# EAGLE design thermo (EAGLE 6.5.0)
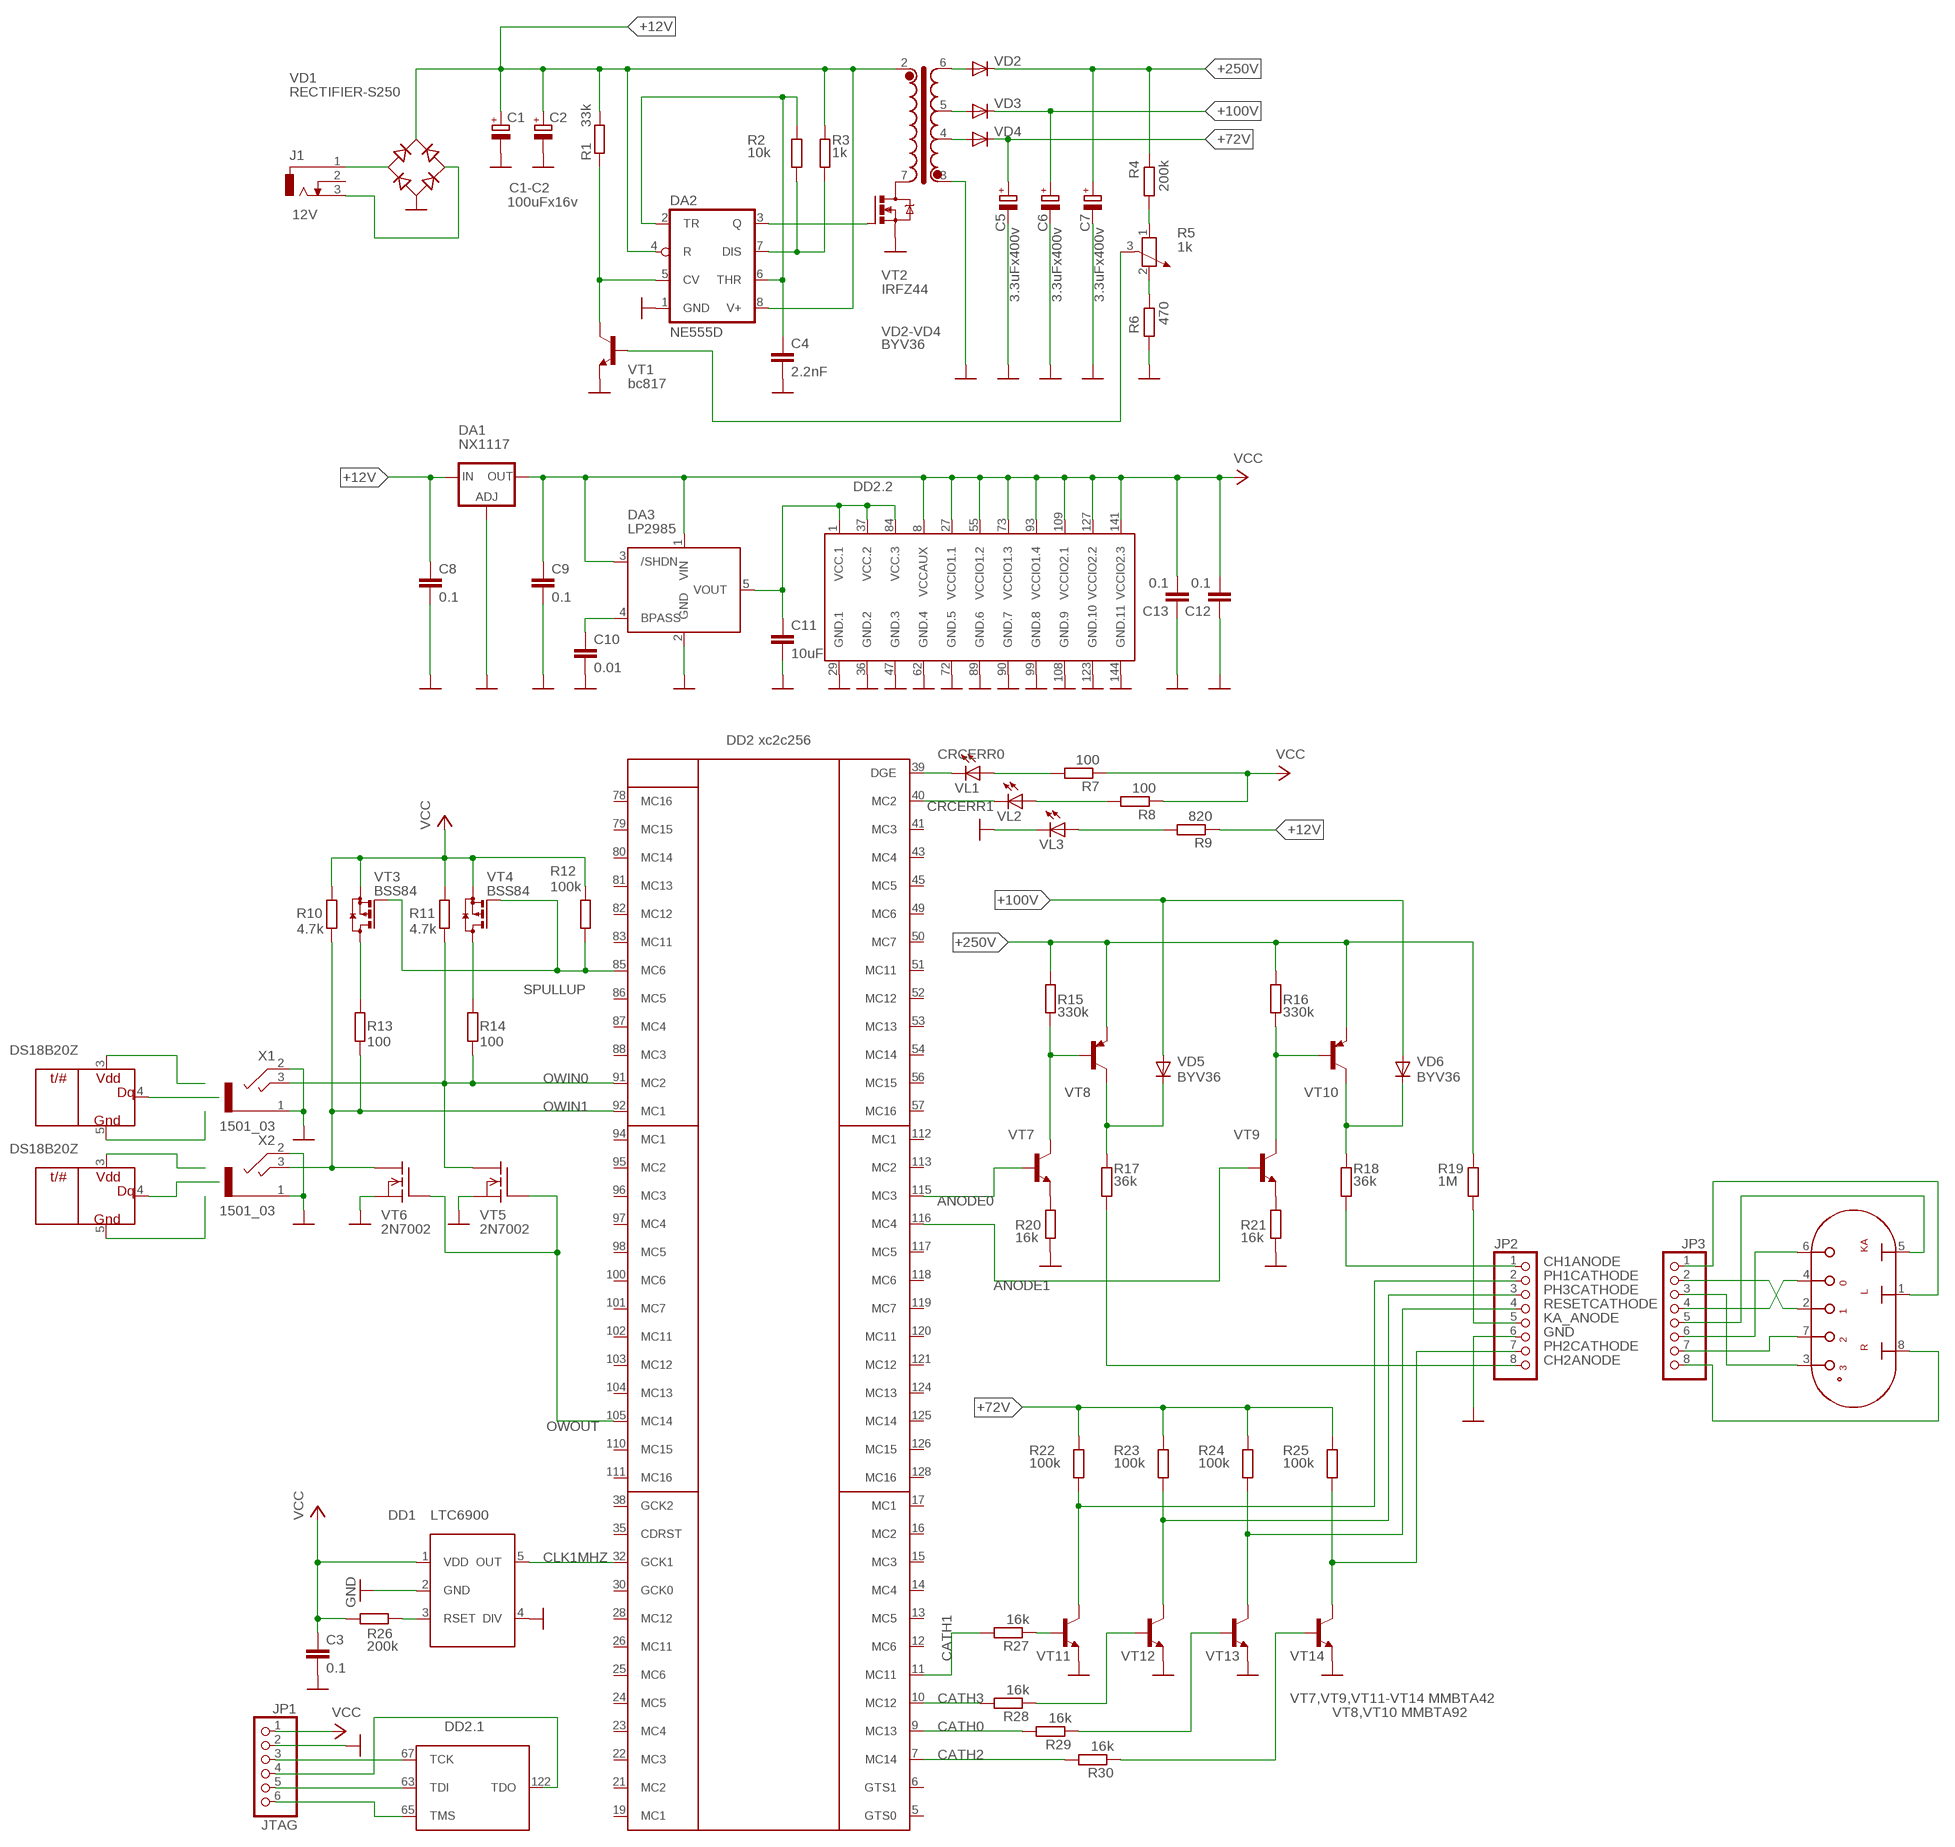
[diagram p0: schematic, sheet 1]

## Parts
C1  100uFx16v  CPOL-EUD  [PANASONIC_D]
C2  100uFx16v  CPOL-EUD  [PANASONIC_D]
C3  0.1  C-EUC1206  [C1206]
C4  2.2nF  C-EUC1206  [C1206]
C5  3.3uFx400v  CPOL-EUE5-10.5  [E5-10,5]
C6  3.3uFx400v  CPOL-EUE5-10.5  [E5-10,5]
C7  3.3uFx400v  CPOL-EUE5-10.5  [E5-10,5]
C8  0.1  C-EUC1206  [C1206]
C9  0.1  C-EUC1206  [C1206]
C10  0.01  C-EUC1206  [C1206]
C11  10uF  C-EUC1206  [C1206]
C12  0.1  C-EUC1206  [C1206]
C13  0.1  C-EUC1206  [C1206]
DA1  NX1117  LD117AS33TR  [SOT223]
DA2  NE555D  [SO08]
DA3  LP2985  [SOT23-5]
DD1  LTC6900  [SOT23-5]
DD2  XC2C128  [TQ144]
J1  DCJ0303  [DCJ0303]
JP1  PINHD-1X6  [1X06]
JP2  PINHD-1X8  [1X08]
JP3  PINHD-1X8  [1X08]
R1  33k  R-EU_R1206  [R1206]
R2  10k  R-EU_R1206  [R1206]
R3  1k  R-EU_R1206  [R1206]
R4  200k  R-EU_R1206  [R1206]
R5  1k  POTENTIOMETER_PT-10  [PT-10]
R6  470  R-EU_R1206  [R1206]
R7  100  R-EU_R1206  [R1206]
R8  100  R-EU_R1206  [R1206]
R9  820  R-EU_R1206  [R1206]
R10  4.7k  R-EU_R1206  [R1206]
R11  4.7k  R-EU_R1206  [R1206]
R12  100k  R-EU_R1206  [R1206]
R13  100  R-EU_R1206  [R1206]
R14  100  R-EU_R1206  [R1206]
R15  330k  R-EU_R1206  [R1206]
R16  330k  R-EU_R1206  [R1206]
R17  36k  R-EU_R1206  [R1206]
R18  36k  R-EU_R1206  [R1206]
R19  1M  R-EU_R1206  [R1206]
R20  16k  R-EU_R1206  [R1206]
R21  16k  R-EU_R1206  [R1206]
R22  100k  R-EU_R1206  [R1206]
R23  100k  R-EU_R1206  [R1206]
R24  100k  R-EU_R1206  [R1206]
R25  100k  R-EU_R1206  [R1206]
R26  200k  R-EU_R1206  [R1206]
R27  16k  R-EU_R1206  [R1206]
R28  16k  R-EU_R1206  [R1206]
R29  16k  R-EU_R1206  [R1206]
R30  16k  R-EU_R1206  [R1206]
T1  TRANSFORM-1  [EFD20-8]
U$2  BG12201  [BG12201]
U$3  DS18B20Z  [SO08]
U$4  DS18B20Z  [SO08]
VD1  RECTIFIER-S250  [TO-269AA]
VD2  BYV36  [SOD57-10]
VD3  BYV36  [SOD57-10]
VD4  BYV36  [SOD57-10]
VD5  BYV36  [SOD57-10]
VD6  BYV36  [SOD57-10]
VL1  LEDCHIPLED_0805  [CHIPLED_0805]
VL2  LEDCHIPLED_0805  [CHIPLED_0805]
VL3  LEDCHIPLED_0805  [CHIPLED_0805]
VT1  bc817  MMBTA42LT1-NPN-SOT23-BEC  [SOT23-BEC]
VT2  IRFZ44  IRFZ48Z  [TO220BH]
VT3  BSS84  [SOT23]
VT4  BSS84  [SOT23]
VT5  2N7002  [SOT23]
VT6  2N7002  [SOT23]
VT7  mmbta42  MMBTA42LT1-NPN-SOT23-BEC  [SOT23-BEC]
VT8  mmbta92  MMBTA92LT1-PNP-SOT23-BEC  [SOT23-BEC]
VT9  mmbta42  MMBTA42LT1-NPN-SOT23-BEC  [SOT23-BEC]
VT10  mmbta92  MMBTA92LT1-PNP-SOT23-BEC  [SOT23-BEC]
VT11  mmbta42  MMBTA42LT1-NPN-SOT23-BEC  [SOT23-BEC]
VT12  mmbta42  MMBTA42LT1-NPN-SOT23-BEC  [SOT23-BEC]
VT13  mmbta42  MMBTA42LT1-NPN-SOT23-BEC  [SOT23-BEC]
VT14  mmbta42  MMBTA42LT1-NPN-SOT23-BEC  [SOT23-BEC]
X1  1501_03  [1501_03]
X2  1501_03  [1501_03]

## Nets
+12V: C1.+ C2.+ C8.1 DA1.3(IN) DA2.4(R) DA2.8(V+) R1.1 R3.1 R9.1 T1.2 VD1.+
+72V: C5.+ R22.2 R23.2 R24.2 R25.2 VD4.C
+100V: C6.+ VD3.C VD5.A VD6.A
+250V: C7.+ R4.1 R15.2 R16.2 R19.2 VD2.C VT8.E VT10.E
ANODE0: DD2.115(FB7:MC3) VT7.B
ANODE1: DD2.116(FB7:MC4) VT9.B
CATH0: DD2.9(FB1:MC13) R29.2
CATH1: DD2.11(FB1:MC11) R27.2
CATH2: DD2.7(FB1:MC14) R30.2
CATH3: DD2.10(FB1:MC12) R28.2
CH1ANODE: JP2.1 R18.1
CH2ANODE: JP2.8 R17.1
CLK1MHZ: DD1.5(OUT) DD2.32(FB2:GCK1)
CRCERR0: DD2.39(FB4:DGE) VL1.C
CRCERR1: DD2.40(FB4:MC2) VL2.C
GND: C1.- C2.- C3.2 C4.2 C5.- C6.- C7.- C8.2 C9.2 C10.2 C11.2 C12.1 C13.1 DA1.1(ADJ) DA2.1(GND) DA3.2(GND) DD1.2(GND) DD1.4(DIV) DD2.29(PWR:GND.1) DD2.36(PWR:GND.2) DD2.47(PWR:GND.3) DD2.62(PWR:GND.4) DD2.72(PWR:GND.5) DD2.89(PWR:GND.6) DD2.90(PWR:GND.7) DD2.99(PWR:GND.8) DD2.108(PWR:GND.9) DD2.123(PWR:GND.10) DD2.144(PWR:GND.11) JP1.2 JP2.6 R6.2 R20.1 R21.1 T1.3 VD1.- VL3.C VT1.E VT2.S VT5.2(S) VT6.2(S) VT11.E VT12.E VT13.E VT14.E X1.1 X1.2 X2.1 X2.2
KA_ANODE: JP2.5 R19.1
N$1: DD1.3(RSET) R26.1
N$2: JP3.1 U$2.1(LA)
N$3: JP3.2 U$2.2(C1)
N$4: C11.1 DA3.5(VOUT) DD2.1(PWR:VCC.1) DD2.37(PWR:VCC.2) DD2.84(PWR:VCC.3)
N$5: JP3.3 U$2.3(C3)
N$6: C10.1 DA3.4(BPASS)
N$7: R20.2 VT7.E
N$8: R21.2 VT9.E
N$9: R15.1 VT7.C VT8.B
N$10: DA2.3(Q) VT2.G
N$11: R16.1 VT9.C VT10.B
N$12: JP3.4 U$2.4(CR)
N$13: JP3.5 U$2.5(KA_A)
N$14: JP3.6 U$2.6(KA_C)
N$15: JP3.7 U$2.7(C2)
N$16: T1.7 VT2.D
N$17: R27.1 VT11.B
N$18: R28.1 VT12.B
N$19: R29.1 VT13.B
N$20: R30.1 VT14.B
N$21: R17.2 VD5.C VT8.C
N$22: R18.2 VD6.C VT10.C
N$23: C4.1 DA2.2(TR) DA2.6(THR) R2.1
N$24: DA2.7(DIS) R2.2 R3.2
N$25: R14.2 VT4.3(D)
N$26: T1.6 VD2.A
N$27: DA2.5(CV) R1.2 VT1.C
N$28: R5.3 VT1.B
N$29: T1.5 VD3.A
N$30: T1.4 VD4.A
N$31: JP3.8 U$2.8(RA)
N$32: U$4.4(DQ)
N$33: U$4.3(VDD)
N$34: DD2.67(JTAG:TCK) JP1.3
N$35: DD2.122(JTAG:TDO) JP1.4
N$36: DD2.63(JTAG:TDI) JP1.5
N$37: DD2.65(JTAG:TMS) JP1.6
N$38: R5.2 R6.1
N$39: R4.2 R5.1
N$40: U$4.5(GND)
N$41: U$3.5(GND)
N$42: J1.1 VD1.AC1
N$43: J1.3 VD1.AC2
N$44: R13.2 VT3.3(D)
N$45: U$3.4(DQ)
N$46: U$3.3(VDD)
N$53: R7.2 VL1.A
N$54: R8.2 VL2.A
N$56: R9.2 VL3.A
OWIN0: DD2.91(FB6:MC2) R11.1 R14.1 VT5.3(D) X1.3
OWIN1: DD2.92(FB6:MC1) R10.1 R13.1 VT6.3(D) X2.3
OWOUT: DD2.105(FB5:MC14) VT5.1(G) VT6.1(G)
PH1CATHODE: JP2.2 R22.1 VT11.C
PH2CATHODE: JP2.7 R25.1 VT14.C
PH3CATHODE: JP2.3 R23.1 VT12.C
RESETCATHODE: JP2.4 R24.1 VT13.C
SPULLUP: DD2.85(FB6:MC6) R12.1 VT3.1(G) VT4.1(G)
VCC: C3.1 C9.1 C12.2 C13.2 DA1.4(OUT) DA3.1(VIN) DA3.3(/SHDN) DD1.1(VDD) DD2.8(PWR:VCCAUX) DD2.27(PWR:VCCIO1.1) DD2.55(PWR:VCCIO1.2) DD2.73(PWR:VCCIO1.3) DD2.93(PWR:VCCIO1.4) DD2.109(PWR:VCCIO2.1) DD2.127(PWR:VCCIO2.2) DD2.141(PWR:VCCIO2.3) JP1.1 R7.1 R8.1 R10.2 R11.2 R12.2 R26.2 VT3.2(S) VT4.2(S)
Unconnected: DD2.2(FB3:GTS2) DD2.3(FB3:GTS3) DD2.4(FB3:MC1) DD2.5(FB1:GTS0) DD2.6(FB1:GTS1) DD2.12(FB1:MC6) DD2.13(FB1:MC5) DD2.14(FB1:MC4) DD2.15(FB1:MC3) DD2.16(FB1:MC2) DD2.17(FB1:MC1) DD2.19(FB2:MC1) DD2.21(FB2:MC2) DD2.22(FB2:MC3) DD2.23(FB2:MC4) DD2.24(FB2:MC5) DD2.25(FB2:MC6) DD2.26(FB2:MC11) DD2.28(FB2:MC12) DD2.30(FB2:GCK0) DD2.35(FB2:CDRST) DD2.38(FB2:GCK2) DD2.41(FB4:MC3) DD2.43(FB4:MC4) DD2.45(FB4:MC5) DD2.49(FB4:MC6) DD2.50(FB4:MC7) DD2.51(FB4:MC11) DD2.52(FB4:MC12) DD2.53(FB4:MC13) DD2.54(FB4:MC14) DD2.56(FB4:MC15) DD2.57(FB4:MC16) DD2.58(FB8:MC16) DD2.59(FB8:MC15) DD2.60(FB8:MC14) DD2.61(FB8:MC13) DD2.64(FB8:MC12) DD2.68(FB8:MC11) DD2.69(FB8:MC6) DD2.70(FB8:MC5) DD2.71(FB8:MC4) DD2.74(FB8:MC3) DD2.76(FB8:MC2) DD2.77(FB8:MC1) DD2.78(FB6:MC16) DD2.79(FB6:MC15) DD2.80(FB6:MC14) DD2.81(FB6:MC13) DD2.82(FB6:MC12) DD2.83(FB6:MC11) DD2.86(FB6:MC5) DD2.87(FB6:MC4) DD2.88(FB6:MC3) DD2.94(FB5:MC1) DD2.95(FB5:MC2) DD2.96(FB5:MC3) DD2.97(FB5:MC4) DD2.98(FB5:MC5) DD2.100(FB5:MC6) DD2.101(FB5:MC7) DD2.102(FB5:MC11) DD2.103(FB5:MC12) DD2.104(FB5:MC13) DD2.110(FB5:MC15) DD2.111(FB5:MC16) DD2.112(FB7:MC1) DD2.113(FB7:MC2) DD2.117(FB7:MC5) DD2.118(FB7:MC6) DD2.119(FB7:MC7) DD2.120(FB7:MC11) DD2.121(FB7:MC12) DD2.124(FB7:MC13) DD2.125(FB7:MC14) DD2.126(FB7:MC15) DD2.128(FB7:MC16) DD2.129(FB3:MC16) DD2.130(FB3:MC15) DD2.131(FB3:MC14) DD2.132(FB3:MC13) DD2.133(FB3:MC12) DD2.134(FB3:MC11) DD2.136(FB3:MC7) DD2.138(FB3:MC6) DD2.140(FB3:MC5) DD2.143(FB3:GSR) J1.2

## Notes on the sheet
- C1-C2
- 12V
- VD2-VD4
- DD2.2
- DD2 xc2c256
- DD1 | LTC6900
- VT7,VT9,VT11-VT14 MMBTA42
- VT8,VT10 MMBTA92
- DD2.1
- JTAG

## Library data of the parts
C1 C2 C5-C7 = rcl:CPOL-EU: POLARIZED CAPACITOR, European symbol
C3 C4 C8-C10 C12 C13 = rcl:C-EU: CAPACITOR, European symbol
C11 = rcl:C-EU: CAPACITOR, European symbol; ESR: 10-20mOhm
DA1 = v-reg:LD117A?*: Low drop fixed and adjustable positive voltage regulators 1 A Source: http://www.st.com/stonline/products/literature/ds/7194/ld1117axx.pdf
DA2 = linear:*555: TIMER
DA3 = coolrunner:LP2985
DD1 = coolrunner:LTC6900
DD2 = coolrunner:XC2C128
J1 = con-jack:DCJ0303: DC POWER JACK Source: DCJ0303.pdf; OC_FARNELL: unknown; OC_NEWARK: unknown
JP1 = pinhead:PINHD-1X6: PIN HEADER
JP2 JP3 = pinhead:PINHD-1X8: PIN HEADER
R1-R4 R6-R30 = rcl:R-EU_: RESISTOR, European symbol
R5 = rcl:POTENTIOMETER_: Potentiometer
T1 = nixie_term:TRANSFORM
U$2 = nixie_term:BG12201
U$3 U$4 = nixie_term:DS18B20
VD1 = rectifier:RECTIFIER-: Rectifier
VD2-VD6 = diode:BYV36: DIODE
VL1-VL3 = led:LED: LED
VT1 VT7 VT9 VT11-VT14 = transistor-neu-to92:*-NPN-: NPN Transistror
VT2 = transistor-power:IRFZ48: N Channel HEXFET® Power MOSFET Logic Level Source: http://www.irf.com/product-info/datasheets/data/irfz48z.pdf
VT3 VT4 = transistor-small-signal:BSS84: P-CHANNEL MOS FET
VT5 VT6 = battery:2N7002
VT8 VT10 = transistor-neu-to92:*-PNP-: PNP Transistror
X1 X2 = con-lumberg:1501_03: Klinkensteckverbinder nach JISC 6560, 2,5 mm Jack connectors according to JISC 6560, 2.5 mm Source: http://www.lumberg.com/Produkte/PDFs/1501_03.pdf; OC_FARNELL: 1200127; OC_NEWARK: unknown

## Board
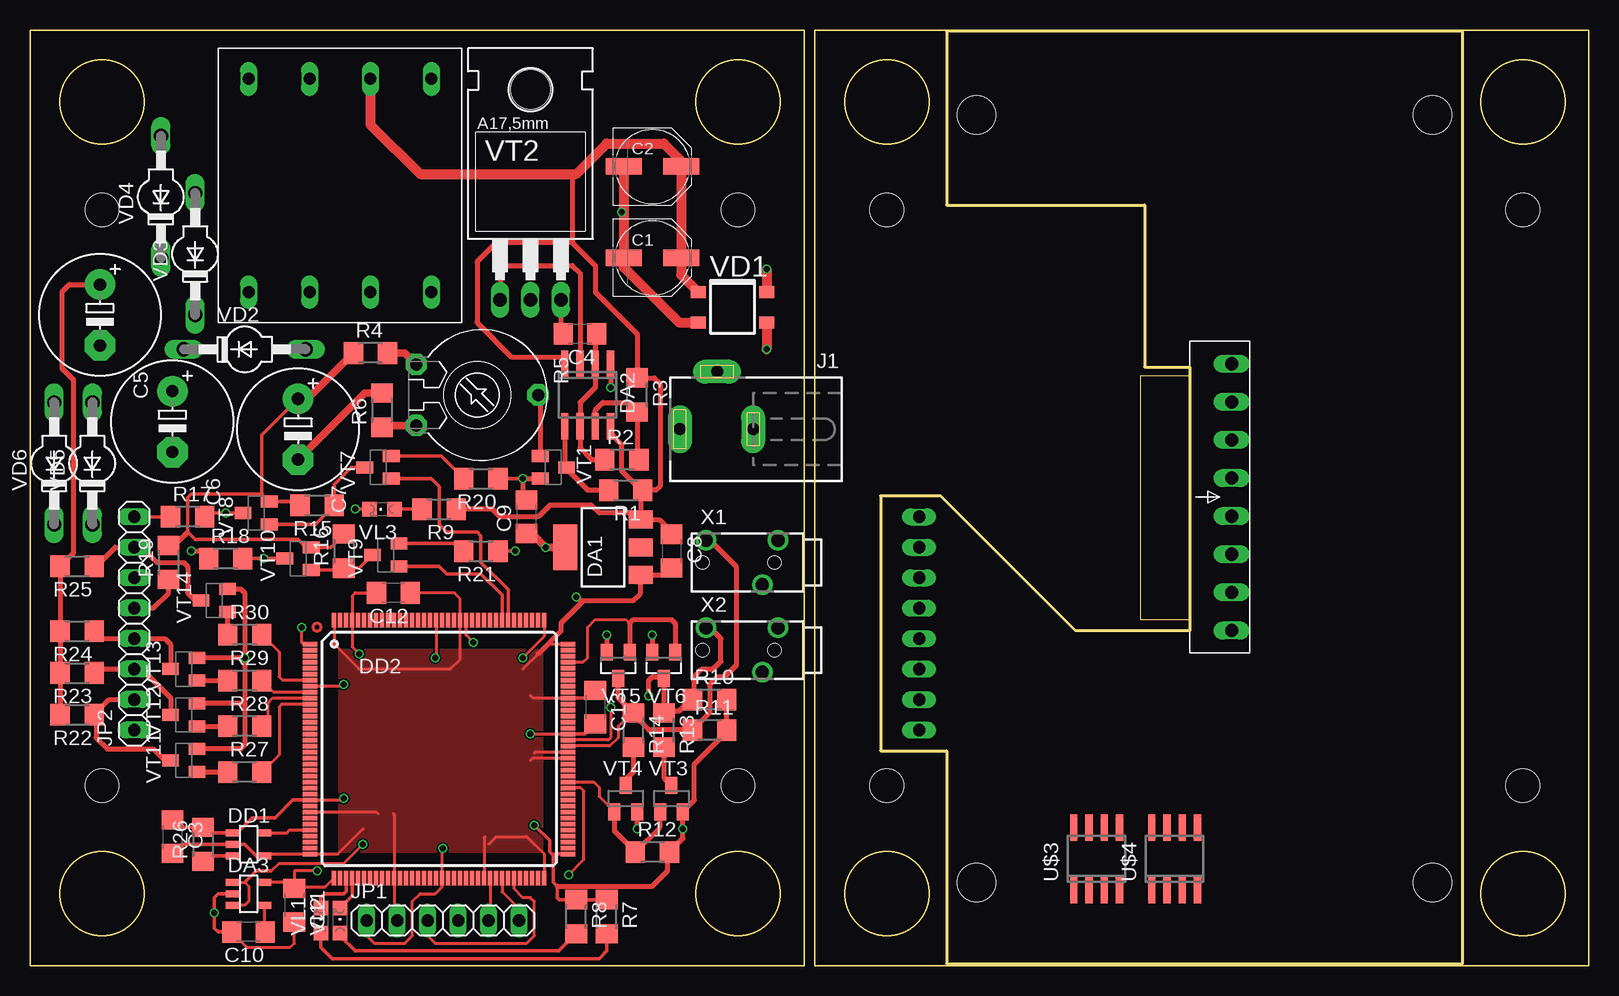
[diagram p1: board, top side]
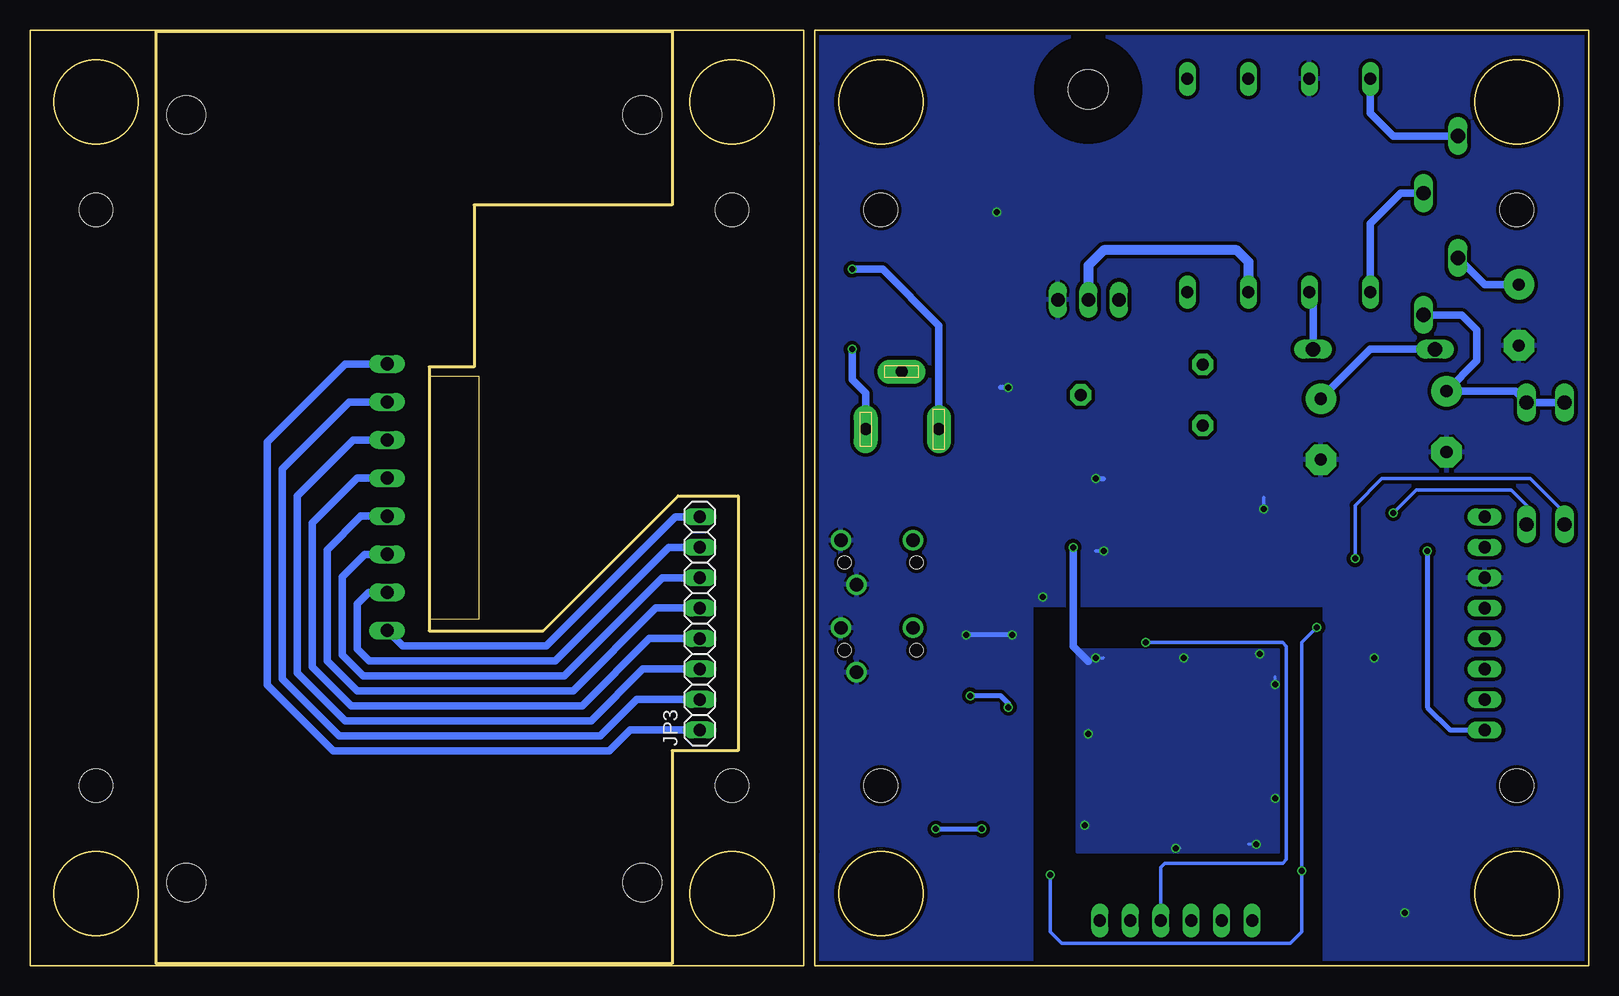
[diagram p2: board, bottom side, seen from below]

Size 129.9 x 78 mm. Coordinates in mm from the lower left corner, seen from the top.
Outline: 70.89,39.15 70.89,17.9 76.39,17.9 76.39,0.15 119.39,0.15 119.39,77.9 76.39,77.9 76.39,63.4 92.89,63.4 92.89,49.9 96.64,49.9 96.64,27.9 87.14,27.9 75.89,39.15 70.89,39.15
Copper layers (1*16): Top 0.035mm / dielectric 1.5mm / Bottom 0.035mm
Design rules "PCB-POOL HighSpec *": minimum track width 0.125mm, minimum drill 0.2mm, track to track 0.125mm, track to pad 0.125mm, pad to pad 0.125mm, via to via 0.125mm, smd to smd 0.125mm, copper to edge 0.3mm, drill to drill 0.2mm, minimum pad ring 0.2mm, minimum via ring 0.125mm, stop-mask expansion 0.075mm, vias tented up to drill 0mil, thermal gap 0.2mm
Holes 3.2 mm at 116.89,70.9 78.89,70.9 78.89,6.9 116.89,6.9

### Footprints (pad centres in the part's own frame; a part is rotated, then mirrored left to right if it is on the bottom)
PANASONIC_D = smd 3 x 1.4: + 2.4,0; - -2.4,0
C1206 = smd 1.6 x 1.8: 1 -1.4,0; 2 1.4,0
E5-10,5 = drill 1.016 pad 2.54: + -2.54,0 | drill 1.016 pad 2.54 octagon: - 2.54,0
SOT223 = smd 1.5 x 2: 1 -2.3,-3.15; 2 0,-3.15; 3 2.3,-3.15 | smd 3.8 x 2: 4 0,3.15
SO08 = smd 0.6 x 2.2: 1 -1.905,-2.6; 2 -0.635,-2.6; 3 0.635,-2.6; 4 1.905,-2.6; 5 1.905,2.6; 6 0.635,2.6; 7 -0.635,2.6; 8 -1.905,2.6
SOT23-5 = smd 0.6 x 1.2: 1 -0.95,-1.306; 2 0,-1.306; 3 0.95,-1.306; 4 0.95,1.306; 5 -0.95,1.306
TQ144 = smd 1.2 x 0.35: 1 -10.75,8.75; 2 -10.75,8.25; 3 -10.75,7.75; 4 -10.75,7.25; 5 -10.75,6.75; 6 -10.75,6.25; 7 -10.75,5.75; 8 -10.75,5.25; 9 -10.75,4.75; 10 -10.75,4.25; 11 -10.75,3.75; 12 -10.75,3.25; 13 -10.75,2.75; 14 -10.75,2.25; 15 -10.75,1.75; 16 -10.75,1.25; 17 -10.75,0.75; 18 -10.75,0.25; 19 -10.75,-0.25; 20 -10.75,-0.75; 21 -10.75,-1.25; 22 -10.75,-1.75; 23 -10.75,-2.25; 24 -10.75,-2.75; 25 -10.75,-3.25; 26 -10.75,-3.75; 27 -10.75,-4.25; 28 -10.75,-4.75; 29 -10.75,-5.25; 30 -10.75,-5.75; 31 -10.75,-6.25; 32 -10.75,-6.75; 33 -10.75,-7.25; 34 -10.75,-7.75; 35 -10.75,-8.25; 36 -10.75,-8.75; 73 10.75,-8.75; 74 10.75,-8.25; 75 10.75,-7.75; 76 10.75,-7.25; 77 10.75,-6.75; 78 10.75,-6.25; 79 10.75,-5.75; 80 10.75,-5.25; 81 10.75,-4.75; 82 10.75,-4.25; 83 10.75,-3.75; 84 10.75,-3.25; 85 10.75,-2.75; 86 10.75,-2.25; 87 10.75,-1.75; 88 10.75,-1.25; 89 10.75,-0.75; 90 10.75,-0.25; 91 10.75,0.25; 92 10.75,0.75; 93 10.75,1.25; 94 10.75,1.75; 95 10.75,2.25; 96 10.75,2.75; 97 10.75,3.25; 98 10.75,3.75; 99 10.75,4.25; 100 10.75,4.75; 101 10.75,5.25; 102 10.75,5.75; 103 10.75,6.25; 104 10.75,6.75; 105 10.75,7.25; 106 10.75,7.75; 107 10.75,8.25; 108 10.75,8.75 | smd 0.35 x 1.2: 37 -8.75,-10.75; 38 -8.25,-10.75; 39 -7.75,-10.75; 40 -7.25,-10.75; 41 -6.75,-10.75; 42 -6.25,-10.75; 43 -5.75,-10.75; 44 -5.25,-10.75; 45 -4.75,-10.75; 46 -4.25,-10.75; 47 -3.75,-10.75; 48 -3.25,-10.75; 49 -2.75,-10.75; 50 -2.25,-10.75; 51 -1.75,-10.75; 52 -1.25,-10.75; 53 -0.75,-10.75; 54 -0.25,-10.75; 55 0.25,-10.75; 56 0.75,-10.75; 57 1.25,-10.75; 58 1.75,-10.75; 59 2.25,-10.75; 60 2.75,-10.75; 61 3.25,-10.75; 62 3.75,-10.75; 63 4.25,-10.75; 64 4.75,-10.75; 65 5.25,-10.75; 66 5.75,-10.75; 67 6.25,-10.75; 68 6.75,-10.75; 69 7.25,-10.75; 70 7.75,-10.75; 71 8.25,-10.75; 72 8.75,-10.75; 109 8.75,10.75; 110 8.25,10.75; 111 7.75,10.75; 112 7.25,10.75; 113 6.75,10.75; 114 6.25,10.75; 115 5.75,10.75; 116 5.25,10.75; 117 4.75,10.75; 118 4.25,10.75; 119 3.75,10.75; 120 3.25,10.75; 121 2.75,10.75; 122 2.25,10.75; 123 1.75,10.75; 124 1.25,10.75; 125 0.75,10.75; 126 0.25,10.75; 127 -0.25,10.75; 128 -0.75,10.75; 129 -1.25,10.75; 130 -1.75,10.75; 131 -2.25,10.75; 132 -2.75,10.75; 133 -3.25,10.75; 134 -3.75,10.75; 135 -4.25,10.75; 136 -4.75,10.75; 137 -5.25,10.75; 138 -5.75,10.75; 139 -6.25,10.75; 140 -6.75,10.75; 141 -7.25,10.75; 142 -7.75,10.75; 143 -8.25,10.75; 144 -8.75,10.75
DCJ0303 = drill 1 pad 2 long: 1 0,3.1; 2 4.8,0; 3 0,-3
1X06 = drill 1.016 long: 1 -6.35,0; 2 -3.81,0; 3 -1.27,0; 4 1.27,0; 5 3.81,0; 6 6.35,0
1X08 = drill 1.016 long: 1 -8.89,0; 2 -6.35,0; 3 -3.81,0; 4 -1.27,0; 5 1.27,0; 6 3.81,0; 7 6.35,0; 8 8.89,0
R1206 = smd 1.6 x 1.803: 1 -1.422,0; 2 1.422,0
PT-10 = drill 1.016 pad 1.778 octagon: 1 -2.54,-5.08; 2 2.54,-5.08; 3 0,5.08
EFD20-8 = drill 1 long: 1 -8.89,7.62; 2 -8.89,2.54; 3 -8.89,-2.54; 4 -8.89,-7.62; 5 8.89,-7.62; 6 8.89,-2.54; 7 8.89,2.54; 8 8.89,7.62
50-200-11 = hole 2.8: -24,-26.5; 24,-26.5; 24,26.5; -24,26.5
BG12201 = drill 1.1 long: 1 11.113,0; 2 7.938,0; 3 4.763,0; 4 1.587,0; 5 -1.587,0; 6 -4.763,0; 7 -7.938,0; 8 -11.113,0
TO-269AA = smd 1 x 1.25: + -1.28,-2.855; - 1.28,-2.855; AC1 -1.28,2.855; AC2 1.28,2.855
SOD57-10 = drill 1.194 long: A 5.08,0; C -5.08,0
CHIPLED_0805 = smd 1.2 x 1.2: A 0,-1.05; C 0,1.05
SOT23-BEC = smd 1 x 1.4: B -0.95,-1.1; C 0,1.1; E 0.95,-1.1
TO220BH = drill 1.118 long: D 0,-6.35; G -2.54,-6.35; S 2.54,-6.35 | hole 3.302: 0,11.176
SOT23 = smd 1 x 1.4: 1 -0.95,-1.1; 2 0.95,-1.1; 3 0,1.1
1501_03 = drill 1.1 pad 1.7: 1 -1.85,0.3; 2 1.85,-1; 3 -1.85,-5.7 | hole 1.1: 0,0; 0,-6

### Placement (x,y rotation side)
C1  51.87,59 0 top
C2  51.87,66.62 0 top
C3  11.86,10.74 270 top
C4  45.84,52.65 180 top
C5  5.83,54.24 270 top
C6  11.86,45.35 270 top
C7  22.34,44.71 270 top
C8  53.45,34.55 270 top
C9  41.39,37.41 90 top
C10  18.21,2.8 180 top
C11  22.02,5.03 270 top
C12  30.28,31.06 180 top
C13  47.11,21.54 270 top
DA1  47.74,34.87 90 top
DA2  46.47,47.57 180 top
DA3  18.21,5.98 270 top
DD1  18.21,10.11 270 top
DD2  34.09,18.04 0 top
J1  57.27,44.71 90 top
JP1  34.41,3.76 0 top
JP2  8.69,28.52 90 top
JP3  74.09,28.52 90 bottom
R1  49.64,39.63 180 top
R2  49.33,42.17 0 top
R3  50.6,47.57 270 top
R4  28.37,51.06 0 top
R5  37.26,47.57 270 top
R6  29.33,46.3 90 top
R7  48.06,4.07 270 top
R8  45.52,4.07 270 top
R9  34.09,38.05 180 top
R10  56.63,22.17 0 top
R11  56.63,19.63 0 top
R12  51.87,9.47 0 top
R13  52.82,19.63 270 top
R14  50.28,19.63 270 top
R15  23.93,38.37 180 top
R16  26.15,34.55 90 top
R17  13.13,37.41 0 top
R18  16.31,33.92 0 top
R19  11.55,33.6 90 top
R20  37.58,40.59 180 top
R21  37.58,34.55 180 top
R22  3.93,20.9 180 top
R23  3.93,24.39 180 top
R24  3.93,27.89 180 top
R25  3.93,33.28 180 top
R26  14.4,10.11 90 top
R27  17.9,16.14 0 top
R28  17.9,19.95 0 top
R29  17.9,23.76 0 top
R30  17.9,27.57 0 top
T1  25.83,65.03 270 top
U$1  [50-200-11]  97.91,39 270 top
U$2  100.14,39.05 90 top
U$3  88.89,8.9 0 top
U$4  95.39,8.9 0 top
U$5  [50-200-11]  32.5,39 270 top
VD1  58.53,54.88 270 top
VD2  17.9,51.38 0 top
VD3  13.77,59.32 90 top
VD4  10.91,64.08 90 top
VD5  5.2,41.86 90 top
VD6  2.02,41.86 90 top
VL1  24.25,3.76 0 top
VL2  25.83,3.76 0 top
VL3  29.33,38.05 90 top
VT1  43.61,41.54 270 top
VT2  41.71,61.86 0 top
VT3  53.45,13.92 0 top
VT4  49.64,13.92 0 top
VT5  49.01,25.03 180 top
VT6  52.82,25.03 180 top
VT7  29.01,41.54 90 top
VT8  18.85,37.73 90 top
VT9  29.64,34.24 90 top
VT10  22.34,33.92 90 top
VT11  12.82,17.09 90 top
VT12  12.82,20.9 90 top
VT13  12.82,24.71 90 top
VT14  15.36,30.43 90 top
X1  62.03,33.6 270 top
X2  62.03,26.3 270 top

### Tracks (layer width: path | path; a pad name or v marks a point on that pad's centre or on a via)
+12V
  Top 0.406: DA2.8 48.38,44.4 49.33,43.45 49.33,41.22 50.92,39.63 | 50.92,39.63 R1.1 52.19,39.63 52.5,39.95 52.5,48.52 52.03,48.99 R3.1 50.6,52.65 47.11,56.14 47.11,58.37 45.2,60.27 | 50.92,39.63 50.92,37.17 DA1.3 | DA2.4 44.56,50.75 40.12,50.75 37.26,53.6 37.26,58.68 38.85,60.27 45.2,60.27 | 54.27,67.08 C2.+ | 45.2,60.27 45.2,65.67 45.52,65.99 | C8.1 53.45,36.14 52.42,37.17 DA1.3 | R9.1 38.53,38.05 39.17,37.41 42.34,37.41 43.3,38.37 46.79,38.37 47.42,37.73 50.33,37.73 DA1.3
  Top 0.813: C2.+ C1.+ 54.27,57.57 VD1.+ | 54.27,67.08 52.82,68.53 48.06,68.53 45.52,65.99 32.5,65.99 28.37,70.12 T1.2
+72V
  Top 0.406: R22.2 R23.2 R24.2 R25.2 3.61,34.39 3.61,48.84 2.66,49.8 2.66,56.14 3.29,56.78 C5.+
  Bottom 0.61: C5.+ 8.69,56.78 VD4.C
+100V
  Bottom 0.61: VD3.C 10.59,54.24 9.32,52.97 9.32,50.43 C6.+ 6.15,47.89 VD5.A VD6.A
+250V
  Top 0.305: R15.2 22.19,38.68 VT8.E 19.31,39.32 | 26,35.82 R16.2 25.04,34.87 VT10.E 22.98,34.87 22.34,35.51 13.77,35.51 13.13,36.14 13.13,39 13.45,39.32 19.31,39.32 | 19.31,39.32 19.31,44.23 C7.+
  Top 0.406: R19.2 12.02,35.02 13.13,36.14
  Top 0.61: C7.+ 23.14,47.25 R4.1
  Bottom 0.61: VD2.C 18.21,51.38 C7.+
ANODE0
  Top 0.305: DD2.115 39.84,31.34 37.58,33.6 37.58,35.82 37.26,36.14 34.72,36.14 34.09,36.78 34.09,39.95 33.45,40.59 VT7.B
ANODE1
  Top 0.305: VT9.B 34.09,33.29 34.72,32.65 37.58,32.65 39.34,30.89 DD2.116
CATH0
  Top 0.254: DD2.9 20.28,22.79 R29.2
CATH1
  Top 0.254: DD2.11 21.01,21.79 20.75,21.54 20.75,17.57 R27.2
CATH2
  Top 0.254: DD2.7 21.04,23.79 20.75,24.08 20.75,26.13 R30.2
CATH3
  Top 0.254: 19.44,20.07 R28.2 19.8,20.43 19.8,21.85 20.24,22.29 DD2.10
CH1ANODE  (via drill 0.5)
  Top 0.406: R18.1 14.89,34.39 14.72,34.55 v13.45,34.55
  Bottom 0.406: v13.45,34.55 13.45,21.54 11.55,19.63 JP2.1
CH2ANODE
  Top 0.305: JP2.8 R17.1
CLK1MHZ
  Top 0.254: DD2.32 21.62,11.29 21.39,11.06 DD1.5
CRCERR0
  Top 0.305: DD2.39 26.34,6.17 26.15,5.98 24.56,5.98 24.25,5.66 VL1.C
CRCERR1
  Top 0.305: DD2.40 26.84,5.81 VL2.C
GND  (via drill 0.5)
  Top 0.254: 30.28,12.65 30.34,12.59 DD2.47 30.34,4.01 JP1.2 | DD2.29 28.86,12.79 29.01,12.65 | 27.74,11.38 25.66,9.29 DD2.36 19.66,9.29 DD1.4 | DD2.144 25.34,26.79 27.42,24.71 35.04,24.71 35.84,25.51 DD2.123 35.84,30.58 35.36,31.06 C12.1 | DD2.108 43.16,26.79 42.34,25.98 41.07,24.71 | DD2.99 41.9,22.29 41.71,22.49 | DD2.89 41.91,17.29 41.71,17.09 | DD2.90 42.09,17.79 42.03,17.73 | DD2.72 42.84,9.29 41.39,10.74 38.85,10.74 38.22,10.11 | DD2.62 37.84,10.68 37.9,10.74 | 16.81,2.93 C10.2 18.08,1.53 21.71,1.53 22.02,1.85 C11.2
  Top 0.305: DD2.99 46.46,22.29 C13.1 | R20.1 v41.07,40.59 | R21.1 v40.44,34.55 | C3.2 12.63,10.11 DD1.2 17.9,10.11 18.85,9.15 DD1.4 | DA3.2 15.67,5.98 15.36,5.66 v15.36,4.39 15.36,3.12 15.67,2.8 C10.2 | VL3.C v27.1,38.05
  Top 0.406: v45.52,30.74 45.84,30.43 46.15,30.43 | 42.34,25.98 44.25,27.89 44.25,28.52 46.15,30.43 | 46.15,30.43 50.28,30.43 50.89,31.04 DA1.1 52.87,32.57 C8.2 | 17.9,29.47 17.89,29.47 | 17.9,29.47 v17.9,25.66 | v17.9,25.66 17.9,21.85 | 17.9,21.85 17.9,18.36 17.58,18.04 VT11.E | VT13.E v17.89,25.66 v17.9,25.66 | VT12.E 17.89,21.85 17.9,21.85 | DA2.1 v48.38,48.21 | C4.2 44.25,52.84 VT2.S | 49.47,62.81 v49.33,62.81 | C1.- 49.47,58.23 | 55.67,53.6 VD1.- | VT6.2 v51.87,27.57 | v48.06,27.57 VT5.2 | VT1.E v41.08,40.59 v41.07,40.59 41.07,39.13 C9.2 | VT14.E 17.58,31.38 17.9,31.06 17.9,29.47
  Top 0.61: R6.2 27.89,47.73 C7.-
  Top 0.813: C2.- 49.47,62.81 C1.- | 49.47,58.23 54.09,53.6 55.67,53.6
  Bottom 0.305: v40.44,34.55 41.07,34.55 | v27.1,38.05 27.1,39
  Bottom 0.406: v48.38,48.21 49.01,48.21 | v48.06,27.57 v51.87,27.57 | v41.07,40.59 40.44,40.59
  pour Top: 42.66,26.3 42.66,9.47 25.83,9.47 25.83,26.3
  pour Bottom (isolate 0.305): 64.25,78.05 64.25,0.26 46.47,0.26 46.47,30.11 22.02,30.11 22.02,-0.05 0.12,-0.05 0.12,78.05
KA_ANODE
  Top 0.406: R19.1 11.55,31.06 10.28,29.79 JP2.5
N$1
  Top 0.305: DD1.3 14.87,9.16 R26.1
N$2
  Bottom 0.61: JP3.1 79.9,19.63 81.64,17.9 104.64,17.9 110.14,23.4 110.14,43.65 103.64,50.15 103.37,50.16 U$2.1
N$3
  Bottom 0.61: JP3.2 79.36,22.17 82.39,19.15 104.14,19.15 108.89,23.9 108.89,41.4 103.3,46.99 U$2.2
N$4  (via drill 0.5)
  Top 0.254: C11.1 22.16,6.57 24.61,6.57 DD2.37 | DA3.5 21.52,6.93 C11.1 | v23.93,7.88 22.02,7.88 C11.1 | DD2.84 45.91,14.79 46.15,14.55 46.15,8.84 v44.88,7.57 | DD2.1 22.8,26.79 22.66,26.93 v22.66,28.2
  Bottom 0.305: v22.66,28.2 23.93,26.93 v23.93,7.88 23.93,2.8 24.88,1.85 43.93,1.85 44.88,2.8 v44.88,7.57
N$5
  Bottom 0.61: JP3.3 78.82,24.71 83.14,20.4 103.64,20.4 107.64,24.4 107.64,39.15 102.97,43.81 U$2.3
N$6
  Top 0.254: DA3.4 19.52,2.9 C10.1
N$7
  Top 0.305: VT7.E 34.25,42.49 R20.2
N$8
  Top 0.305: VT9.E 35.53,35.19 R21.2
N$9
  Top 0.305: VT8.B 23.77,36.78 R15.1 25.35,40.1 26.79,41.54 VT7.C
N$10
  Top 0.406: DA2.3 45.84,57.73 45.2,58.37 39.48,58.37 39.17,58.05 VT2.G
N$11
  Top 0.305: VT9.C 27.44,33.13 R16.1 25.99,32.97 VT10.B
N$12
  Bottom 0.61: JP3.4 78.28,27.25 83.89,21.65 103.14,21.65 106.39,24.9 106.39,36.9 102.65,40.64 U$2.4
N$13
  Bottom 0.61: JP3.5 77.74,29.79 84.64,22.9 102.64,22.9 105.14,25.4 105.14,34.65 102.32,37.46 U$2.5
N$14
  Bottom 0.61: JP3.6 77.2,32.33 85.39,24.15 102.14,24.15 103.89,25.9 103.89,32.4 102,34.29 U$2.6
N$15
  Bottom 0.61: JP3.7 76.66,34.87 86.14,25.4 101.64,25.4 102.64,26.4 102.64,30.15 101.67,31.11 U$2.7
N$16
  Bottom 0.813: VT2.D 41.71,58.37 40.44,59.64 29.33,59.64 28.37,58.68 T1.7
N$17
  Top 0.406: VT11.B R27.1
N$18
  Top 0.406: VT12.B R28.1
N$19
  Top 0.406: VT13.B R29.1
N$20
  Top 0.406: R30.1 16.46,27.59 VT14.B
N$21  (via drill 0.5)
  Top 0.305: VT8.C v16.31,37.73 14.87,37.73 R17.2
  Bottom 0.305: VD5.C 5.2,38.37 6.47,39.63 14.4,39.63 v16.31,37.73
N$22  (via drill 0.5)
  Top 0.305: VT10.C v19.48,33.92 R18.2
  Bottom 0.305: VD6.C 2.02,37.73 4.88,40.59 17.26,40.59 19.48,38.37 v19.48,33.92
N$23
  Top 0.406: R2.1 46.79,42.17 45.84,43.13 DA2.6 45.84,46.94 47.11,48.21 DA2.2 47.11,52.52 C4.1
N$24
  Top 0.406: DA2.7 47.11,46.3 47.74,46.94 49.81,46.94 R3.2 50.6,42.33 R2.2
N$25
  Top 0.406: R14.2 50.28,16.14 49.64,15.5 VT4.3
N$26
  Bottom 0.61: VD2.A 22.98,55.83 T1.6
N$27
  Top 0.406: DA2.5 44.56,41.69 VT1.C 44.71,41.39 46.47,39.63 R1.2
N$28
  Top 0.406: VT1.B 42.51,47.4 R5.3
N$29
  Bottom 0.61: VD3.A 15.67,64.4 18.21,61.86 T1.5
N$30
  Bottom 0.61: VD4.A 16.31,69.16 18.21,71.07 T1.4
N$31
  Bottom 0.61: JP3.8 76.12,37.41 86.89,26.65 98.85,26.65 U$2.8
N$34
  Top 0.254: JP1.3 33.14,2.49 33.77,1.85 41.39,1.85 42.03,2.49 42.03,5.34 41.71,5.66 41.07,5.66 40.34,6.4 DD2.67
N$35  (via drill 0.5)
  Top 0.254: DD2.122 36.34,27.54 v36.95,26.93
  Bottom 0.305: v36.95,26.93 25.52,26.93 25.2,26.62 25.2,8.84 25.52,8.52 35.36,8.52 35.67,8.2 JP1.4
N$36
  Top 0.254: DD2.63 38.34,3.88 JP1.5
N$37
  Top 0.254: DD2.65 39.34,6.13 40.75,4.71 JP1.6
N$38
  Top 0.61: R6.1 29.48,45.03 R5.2
N$39
  Top 0.61: R4.2 31.23,51.06 R5.1
N$42  (via drill 0.5)
  Top 0.406: v61.39,58.05
  Top 0.813: v61.39,58.05 VD1.AC1
  Bottom 0.61: J1.1 54.17,53.36 58.85,58.05 v61.39,58.05
N$43  (via drill 0.5)
  Top 0.406: v61.39,51.38
  Top 0.813: VD1.AC2 v61.39,51.38
  Bottom 0.61: J1.3 60.27,47.71 61.39,48.84 v61.39,51.38
N$44
  Top 0.406: R13.2 52.82,15.65 VT3.3
N$53
  Top 0.305: VL1.A 24.25,1.53 25.2,0.58 47.42,0.58 48.06,1.22 R7.2
N$54
  Top 0.305: VL2.A 25.83,2.49 27.1,1.22 44.08,1.22 R8.2
N$56
  Top 0.305: VL3.A R9.2
OWIN0
  Top 0.254: R14.1 50.11,21.05 49.01,19.95 49.01,19 48.31,18.29 DD2.91
  Top 0.406: X1.3 56.69,35.45 58.85,33.28 58.85,25.03 57.9,24.08 57.27,24.08 56.63,23.44 56.63,21.05 R11.1 51.55,19.63 50.28,20.9 R14.1 49.01,22.32 VT5.3
OWIN1  (via drill 0.5)
  Top 0.254: DD2.92 48.17,18.79 48.38,19 v48.38,21.54
  Top 0.406: X2.3 56.69,28.15 57.58,27.25 57.58,25.35 56.95,24.71 56,24.71 55.36,24.08 55.36,22.32 R10.1 55.04,22.17 54.09,21.22 52.98,21.22 R13.1 VT6.3 52.67,24.08 51.87,24.08 51.55,23.76 v51.55,22.49
  Bottom 0.406: v48.38,21.54 48.38,21.85 49.01,22.49 v51.55,22.49
OWOUT
  Top 0.254: DD2.105 46.1,25.29 46.47,25.66 46.47,28.2 47.11,28.84 49.64,28.84 49.96,28.52
  Top 0.406: VT6.1 53.77,28.52 53.45,28.84 50.28,28.84 49.96,28.52 VT5.1
PH1CATHODE
  Top 0.406: JP2.2 6.62,22.17 R22.1 5.51,20.74 5.51,19 6.47,18.04 10.28,18.04 11.23,17.09 VT11.C
PH2CATHODE
  Top 0.406: VT14.C 13.77,30.43 13.13,31.06 13.13,33.28 12.82,33.6 10.59,33.6 9.32,34.87 JP2.7 7.1,34.87 5.51,33.28 R25.1
PH3CATHODE
  Top 0.406: R23.1 5.66,24.71 JP2.3 9.32,24.71 11.72,22.32 VT12.C
RESETCATHODE
  Top 0.406: R24.1 5.98,27.25 JP2.4 11.23,27.25 11.72,26.76 VT13.C
SPULLUP
  Top 0.254: DD2.85 47,15.29 47.42,14.87 47.42,14.09 VT4.1
  Top 0.406: VT3.1 52.5,11.53 R12.1 48.7,11.22 VT4.1
VCC  (via drill 0.5)
  Top 0.254: DA3.1 | DD2.93 41.73,19.29 v41.71,19.31 | DD2.109 42.84,27.43 v41.07,25.66 | DD2.127 33.84,25.73 v33.77,25.66 | v27.42,25.98 26.84,26.56 DD2.141 26.84,30.8 27.1,31.06 C12.2 | DD2.8 26,23.29 v26.15,23.44 | DD2.27 26.03,13.79 v26.15,13.92 | v34.41,9.79 34.34,9.72 DD2.55 34.34,6.55 33.77,5.98 32.5,5.98 31.87,5.34 31.87,2.49 31.23,1.85 28.69,1.85 28.06,2.49 JP1.1 | 43.47,9.29 DD2.73 | DA3.3 17.9,5.03 18.21,5.34 18.21,6.61 17.9,6.93 DA3.1 | DA3.1 16.62,6.93 | 20.12,7.88 20.75,8.52 26.15,8.52 v27.74,10.11 | 43.75,9.29 43.61,9.15
  Top 0.305: 43.47,9.29 43.3,9.47 43.3,10.42 v42.03,11.69 | 20.12,7.88 18.85,7.88 17.9,6.93 | DD2.73 43.75,9.29 | 43.61,9.15 43.61,6.93 43.93,6.61 43.93,5.66 44.1,5.5 R8.1 R7.1 | DD2.93 46.26,19.29 C13.2 | DD2.27 21.9,13.79 20.44,12.33 18.53,12.33 17.26,11.06 DD1.1 14.87,11.06 R26.2 12.48,11.53 C3.1
  Top 0.406: R10.2 R11.2 58.05,19.47 55.36,16.77 55.36,13.77 VT3.2 v54.41,11.38 54.41,10.59 R12.2 53.14,9.32 53.14,7.88 51.87,6.61 43.93,6.61 | VT4.2 v50.59,11.38 v50.6,11.38
  Top 0.61: DA1.4 v42.98,34.87 41.84,36.01 C9.1
  Bottom 0.254: v41.71,19.31 41.71,19.63 | v41.07,25.66 40.44,25.66 | v33.77,25.66 33.45,25.66 | v27.42,25.98 27.74,25.98 | v26.15,23.44 26.15,24.08 | v26.15,13.92 26.15,14.23 | v34.41,9.79 34.09,9.79 | v42.03,11.69 42.03,12.01 | v27.74,10.11 28.37,10.11
  Bottom 0.406: v54.41,11.38 v50.6,11.38
  Bottom 0.61: v42.98,34.87 42.98,26.62 41.71,25.35
  pour Bottom: 42.66,26.3 42.66,9.47 25.83,9.47 25.83,26.3
(copper drawn outside any net)
  shapes: Top circle x1

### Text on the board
case_top: o | C | 4O | 3O | 2O | 1O | O | -1O | -2O | -3O | -4O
